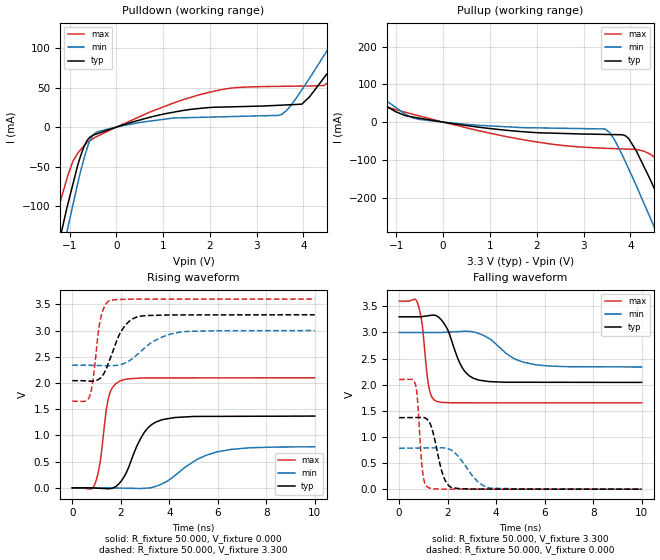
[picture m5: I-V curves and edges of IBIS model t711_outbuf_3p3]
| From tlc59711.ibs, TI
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|   t711_outbuf 3.3V Model
[Model] t711_outbuf_3p3
Model_type   Output
Polarity   Non-Inverting
Vmeas = 1.65
Vref = 1.65
Rref = 50
|   typ   min   max
|   (nom PVT)   (Fast PVT)   (slow PVT)
|   ON state : BUFFER OUTPUT TURNED HIGH
C_comp   2.21861E-12   1.89706E-12   2.43266E-12
|   OFF state: BUFFER OUTPUT TURNED LOW
|C_comp   2.16811E-12   2.08969E-12   2.20842E-12
| Where   nom PVT is  Nominal Process, 3.3V, 90C
|   Fast PVT is Strong Process, 3.6V, -40C
|   Slow PVT is Weak Process, 3.0V, 150C
|   C_comp - from L-C Tank method, L = 1nH, peak frequency
| variable   typ   min   max
[Voltage Range]   3.3   3   3.6
|Operating Temperature Range
|   25   85   -40
|Junction Temperature Range
[Temperature Range]   90   150   -40
[Pullup Reference]   3.3   3   3.6
[Pulldown Reference]   0   0   0
[Power Clamp Reference]   3.3   3   3.6
[GND Clamp Reference]   0   0   0
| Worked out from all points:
|   slope of the pulldown table from 0 to 0.495 V, typ, clamps not added: 55.5 ohm
|   slope of the pullup table from 0 to 0.495 V, typ, clamps not added: 55.1 ohm
|   falling waveform, R_fixture 50.000, V_fixture 3.300: 20-80 % time 639ps typ, 1.11ns min, 262ps max; typ from 3.3 V to 2.04 V
|   rising waveform, R_fixture 50.000, V_fixture 0.000: 20-80 % time 822ps typ, 1.55ns min, 356ps max; typ from 0 V to 1.37 V
|   rising waveform, R_fixture 50.000, V_fixture 3.300: 20-80 % time 685ps typ, 1.16ns min, 310ps max; typ from 2.04 V to 3.3 V
|   falling waveform, R_fixture 50.000, V_fixture 0.000: 20-80 % time 415ps typ, 773ps min, 184ps max; typ from 1.37 V to 0 V
[Pulldown]
|   Voltage   I(typ)   I(min)   I(max)
-3.3V     -720mA     -779.8mA   -630.4mA
-1.468V   -211.3mA   -247.9mA   -153.2mA
-1.061V   -103.6mA   -134.3mA   -66.59mA
-694.2mV  -25.3mA    -40.39mA   -23.96mA
-417.7mV  -8.498mA   -6.2mA     -11.86mA
1.741V    23.47mA    12.34mA    40.46mA
3.499V    27.8mA     15.38mA    51.77mA
3.963V    29.1mA     47.09mA    52.1mA
4.437V    62.48mA    90.76mA    52.75mA
4.909V    99.34mA    134.9mA    80.19mA
5.107V    115.8mA    153.5mA    93.22mA
6.59V     238.7mA    296.2mA    190.7mA
[Pullup]
|   Voltage   I(typ)   I(min)   I(max)
-3.3V     211.2mA    252.6mA    158.1mA
-1.76V    85.54mA    106.3mA    59.14mA
-666.3mV  13.85mA    11.96mA    21.52mA
1.741V    -25.67mA   -14.66mA   -47.38mA
3.466V    -32.6mA    -18.79mA   -69.33mA
3.64V     -33.03mA   -42.71mA   -70.14mA
3.963V    -43.33mA   -123.6mA   -71.64mA
4.289V    -117.5mA   -214.8mA   -76.82mA
4.54V     -183.5mA   -286.6mA   -97.45mA
4.866V    -271.7mA   -379.8mA   -172.2mA
5.2V      -364.9mA   -476.4mA   -258.1mA
6.59V     -753.4mA   -883.4mA   -625.9mA
[Ramp]
R_load = 50
|   typ   min   max
dV/dt_r   0.821245/8.18928e-010   0.47007/1.53918e-009   1.25954/3.54404e-010
dV/dt_f   0.753432/6.37347e-010  0.424782/1.11335e-009   1.16829/2.60909e-010
[Falling Waveform]
R_fixture = 50.000
V_fixture = 3.300
V_fixture_min = 3.000
V_fixture_max = 3.600
C_fixture = 0.000
|  time   V(typ)   V(min)   V(max)
0s        3.3V       3V         3.6V
757.7ps   3.301V     3V         3.566V
952.1ps   3.305V     3V         3.152V
1.227ns   3.323V     3V         1.952V
1.533ns   3.32V      3V         1.683V
2.016ns   3.039V     3.007V     1.657V
2.632ns   2.303V     3.022V     1.654V
3.25ns    2.093V     2.986V     1.653V
5.623ns   2.047V     2.383V     1.653V
10ns      2.044V     2.339V     1.653V
[Rising Waveform]
R_fixture = 50.000
V_fixture = 0.000
V_fixture_min = 0.000
V_fixture_max = 0.000
C_fixture = 0.000
|  time   V(typ)   V(min)   V(max)
0s        29.04uV    9.844uV    94.07uV
914.9ps   -3.018mV   -216.1uV   52.31mV
1.154ns   -8.572mV   -275.2uV   506mV
1.383ns   -13.89mV   -331.7uV   1.417V
1.496ns   -16.53mV   -359.8uV   1.718V
1.993ns   115.3mV    -4.247mV   2.043V
2.965ns   1.054V     -8.038mV   2.096V
3.681ns   1.296V     73.15mV    2.097V
5.967ns   1.363V     685.3mV    2.098V
10ns      1.369V     783.5mV    2.099V
[Rising Waveform]
R_fixture = 50.000
V_fixture = 3.300
V_fixture_min = 3.000
V_fixture_max = 3.600
C_fixture = 0.000
|  time   V(typ)   V(min)   V(max)
0s        2.044V     2.339V     1.653V
728.2ps   2.036V     2.338V     1.761V
864.1ps   2.032V     2.336V     2.087V
1.158ns   2.092V     2.331V     3.207V
1.326ns   2.2V       2.329V     3.456V
1.539ns   2.437V     2.326V     3.572V
2.038ns   3.004V     2.357V     3.594V
2.728ns   3.269V     2.563V     3.599V
4.49ns    3.298V     2.974V     3.599V
10ns      3.3V       3V         3.6V
[Falling Waveform]
R_fixture = 50.000
V_fixture = 0.000
V_fixture_min = 0.000
V_fixture_max = 0.000
C_fixture = 0.000
|  time   V(typ)   V(min)   V(max)
0s        1.369V     783.5mV    2.099V
672.2ps   1.372V     786.9mV    2.004V
760ps     1.373V     787.4mV    1.697V
893.5ps   1.373V     788.1mV    713.9mV
971.7ps   1.374V     788.5mV    321.1mV
1.218ns   1.307V     789.7mV    24.74mV
1.813ns   262mV      790.7mV    698uV
2.174ns   28.9mV     738.1mV    671.8uV
3.764ns   1.281mV    20.41mV    556.7uV
10ns      51.81uV    25.12uV    105.2uV
